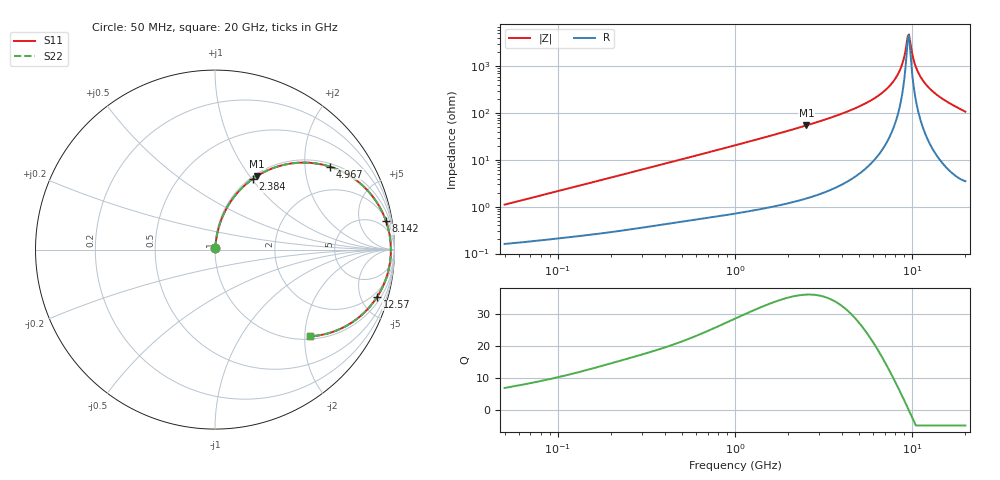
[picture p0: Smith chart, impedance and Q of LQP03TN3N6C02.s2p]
!Murata Part Number: LQP03TN3N6C02
!These Parameters are Measured in Series Mode Connection
!  o--[Z]--o
!Port1  Port2
!  o-------o
!Freq. Start=50[MHz] Stop=20[GHz], 401[Steps]
# Hz S RI R 50
!Freq.(Hz) S11(Real) S11(Imag) S21(Real) S21(Imag) S12(Real) S12(Imag) S22(Real) S22(Imag)
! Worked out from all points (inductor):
!   401 points, 50 MHz to 20 GHz, reference 50 ohm
!   read as one part in series: L = 3.46 nH near 51.52 MHz
!   highest Q = 36.2 at 2.531 GHz (marker M1), where L = 3.42 nH
!   self-resonance near 9.457 GHz
!   S11 on the Smith chart (normalised r, x): 50 MHz: 1.00, +0.02; 2.384 GHz: 1.03, +1.02; 4.967 GHz: 1.10, +2.70; 8.142 GHz: 2, +12; 12.57 GHz: 1.45, -6.64; 20 GHz: 1.07, -2.13
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5e7  0.00172 0.0109  0.9983 -0.0109  0.9983 -0.0109  0.00172 0.0109
1.364002e8  0.00322 0.0288  0.9968 -0.0288  0.9968 -0.0288  0.00322 0.0288
3.721004e8  0.00984 0.0758  0.9902 -0.0758  0.9902 -0.0758  0.00984 0.0758
1e9  0.0463 0.1934  0.9537 -0.1934  0.9537 -0.1934  0.0463 0.1934
2.383959e9  0.2117 0.3949  0.7883 -0.3949  0.7883 -0.3949  0.2117 0.3949
2.531158e9  0.2344 0.41  0.7656 -0.41  0.7656 -0.41  0.2344 0.41
2.728004e9  0.2658 0.4282  0.7342 -0.4282  0.7342 -0.4282  0.2658 0.4282
4.966507e9  0.6413 0.4619  0.3587 -0.4619  0.3587 -0.4619  0.6413 0.4619
6.311513e9  0.8187 0.3603  0.1813 -0.3603  0.1813 -0.3603  0.8187 0.3603
7.442007e9  0.9163 0.2394  0.0837 -0.2394  0.0837 -0.2394  0.9163 0.2394
8.141811e9  0.953 0.1586  0.047 -0.1586  0.047 -0.1586  0.953 0.1586
8.644534e9  0.9693 0.1006  0.0307 -0.1006  0.0307 -0.1006  0.9693 0.1006
8.907419e9  0.9747 0.0707  0.0253 -0.0707  0.0253 -0.0707  0.9747 0.0707
9.316812e9  0.9794 0.0252  0.0206 -0.0252  0.0206 -0.0252  0.9794 0.0252
9.600142e9  0.9801 -0.00542  0.0199 0.00542  0.0199 0.00542  0.9801 -0.00542
9.745021e9  0.9797 -0.0208  0.0203 0.0208  0.0203 0.0208  0.9797 -0.0208
1.019291e10  0.9757 -0.0666  0.0243 0.0666  0.0243 0.0666  0.9757 -0.0666
1.066139e10  0.9674 -0.1119  0.0326 0.1119  0.0326 0.1119  0.9674 -0.1119
1.149051e10  0.9442 -0.1848  0.0558 0.1848  0.0558 0.1848  0.9442 -0.1848
1.257102e10  0.9022 -0.2653  0.0978 0.2653  0.0978 0.2653  0.9022 -0.2653
1.527346e10  0.7693 -0.4017  0.2307 0.4017  0.2307 0.4017  0.7693 -0.4017
2e10  0.531 -0.4829  0.469 0.4829  0.469 0.4829  0.531 -0.4829
